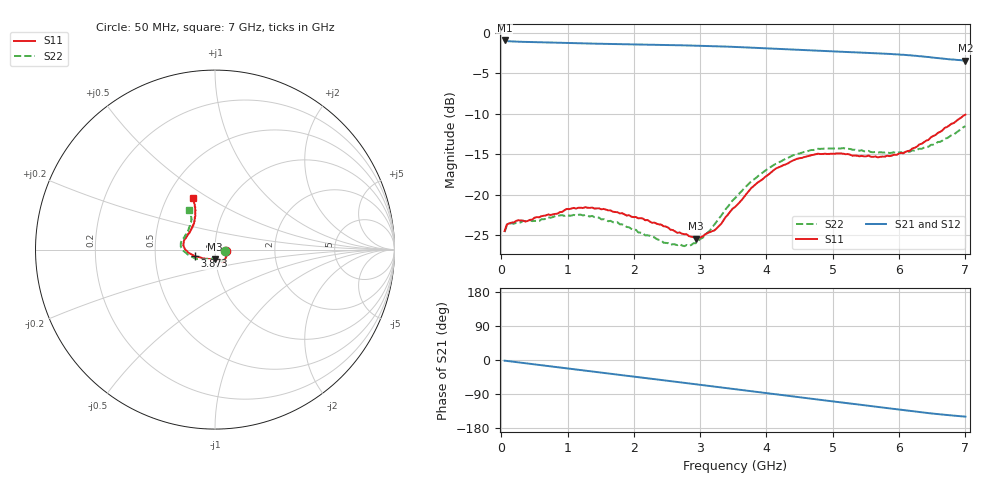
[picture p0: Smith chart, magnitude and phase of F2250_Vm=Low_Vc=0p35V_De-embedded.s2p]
! Integrated Device Technology
! Corporate Headquarters
! 6024 Silver Creek Valley Road
! San Jose, CA 95138  USA
! Phone:  1-408-284-8200
! Toll Free:  1-800-223-1366
! Webpage:  http://www.idt.com/
! Timing and RF Division
! 515 Groton Road, Suite 102
! Westford, MA 01886-6024
! Device:  F2250
! Description: Voltage Variable RF Attenuator
! Frequency:  50.0 -  6000.00 MHz
! Package:  3x3 mm Thin QFN Plastic Package: 16 pin
! Ports:  2 RF, 3 DC
!  Pin  1  = GND
!  Pin  2  = NC
!  Pin  3  = RF1  = Port 1
!  Pin  4  = NC
!  Pin  5  = GND
!  Pin  6  = GND
!  Pin  7  = GND
!  Pin  8  = GND
!  Pin  9  = NC
!  Pin 10  = RF2  = Port 2
!  Pin 11  = NC
!  Pin 12  = GND
!  Pin 13  = GND
!  Pin 14  = VCNTRL
!  Pin 15  = VDD
!  Pin 16  = VMODE
! Vcntrl:  0.350 Volts
! Vmode:  +0.000 Volts
! Vdd:  +3.30  Volts
! Current:  1.119 mA
! Data:  The device was measured on a the F2250 evaluation board which has
!  individual transmission lines to the RF pins.  Data was collected
!  using a calibrated network analyzer.  The evaluation board was
!  de-embedded using a TRL calibration technique.
!  The reference plane is the edge of the package pin.
! Misc:  SN 10
!  Action Tracker AT0258
! Date Measured:  2014-11-26
! Date:  2015-10-15  MJV
! Note:
!  Integrated Device Technology supplies this data as a sample of measured
!  data at the package pin for this product.  Your particular data for this
!  product may vary.
!  Data was taken at 25 degrees C.
!  Integrated Device Technology reserves the right to change this data at anytime.
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# GHz S dB R 50
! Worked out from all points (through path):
!   201 points, 50 MHz to 7 GHz, reference 50 ohm
!   highest |S21| = -0.97 dB at 50 MHz (marker M1); lowest = -3.4 dB at 7 GHz (marker M2)
!   group delay of S21, straight-line fit = 60 ps
!   lowest |S11| = -25.4 dB at 2.934 GHz (marker M3), VSWR 1.11, Z = 49.8 - j5.36 ohm
!   |S11| at or under -10 dB: start of sweep to end of sweep
!   |S22| runs from -26.3 to -11.5 dB; largest |S21 - S12| = 0.00031
!   S11 on the Smith chart (normalised r, x): 50 MHz: 1.13, -0.02; 3.873 GHz: 0.79, -0.06; 7 GHz: 0.67, +0.43
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0.05  -24.47 -9.1  -0.97 -1.8  -0.97 -1.8  -24.60 -9.6
0.08475  -23.65 -9.0  -1.04 -2.5  -1.04 -2.5  -23.73 -9.0
0.15425  -23.43 -11.2  -1.09 -4.0  -1.08 -4.0  -23.50 -10.7
0.57125  -22.78 -28.7  -1.19 -13.1  -1.19 -13.1  -23.24 -29.7
0.884  -22.14 -44.0  -1.25 -19.9  -1.25 -19.9  -22.54 -45.8
1.2315  -21.64 -54.1  -1.33 -27.4  -1.33 -27.4  -22.55 -58.6
1.75275  -22.15 -60.7  -1.42 -38.4  -1.42 -38.4  -23.38 -66.0
2.37825  -23.65 -61.7  -1.51 -51.8  -1.51 -51.8  -25.57 -68.7
2.552  -24.30 -65.7  -1.54 -55.6  -1.54 -55.6  -26.20 -74.4
2.83  -25.10 -80.2  -1.59 -61.7  -1.59 -61.7  -26.31 -92.8
2.93425  -25.41 -88.7  -1.61 -64.0  -1.61 -64.0  -25.97 -101.3
3.21225  -24.40 -117.9  -1.67 -70.2  -1.67 -70.2  -23.68 -126.6
3.525  -21.51 -145.2  -1.77 -77.1  -1.77 -77.1  -20.43 -145.5
3.8725  -18.45 -162.1  -1.90 -84.8  -1.90 -84.8  -17.70 -160.9
4.1505  -16.72 -172.1  -2.01 -90.9  -2.01 -90.9  -16.13 -170.8
4.4285  -15.68 -179.8  -2.12 -96.9  -2.12 -96.9  -15.04 -178.0
4.7065  -15.07 173.5  -2.22 -102.9  -2.22 -102.9  -14.48 176.0
5.15825  -14.94 162.7  -2.38 -112.6  -2.38 -112.6  -14.24 166.7
5.85325  -15.23 139.4  -2.63 -127.5  -2.63 -127.6  -14.85 151.6
6.166  -14.54 128.4  -2.80 -134.4  -2.80 -134.4  -14.68 142.7
6.444  -13.23 120.0  -3.01 -140.1  -3.01 -140.2  -14.07 133.3
7  -10.11 113.5  -3.45 -149.4  -3.45 -149.4  -11.53 123.8
